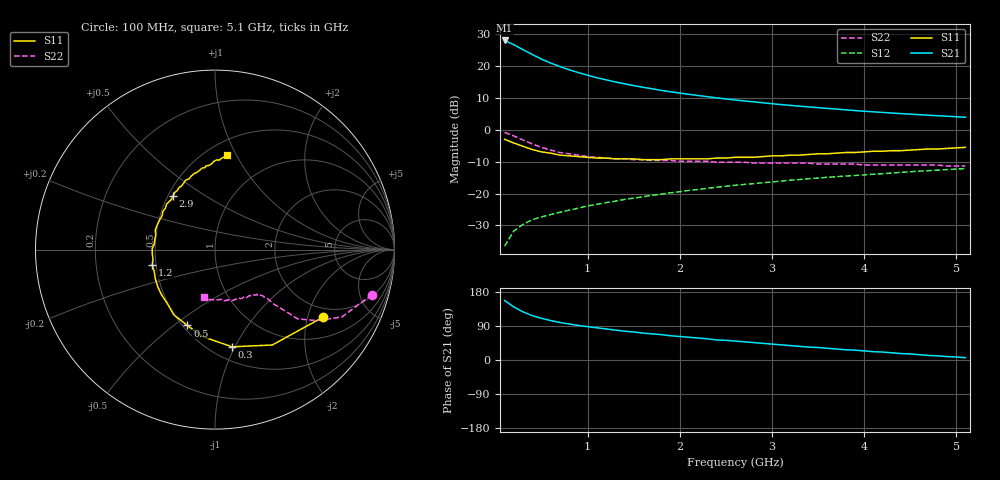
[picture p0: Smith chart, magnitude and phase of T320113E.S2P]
!AT-32011
!S PARAMETERS at Vce=2.7 V  Ic=10mA.  LAST UPDATED 01-05-95
# ghz s ma r 50
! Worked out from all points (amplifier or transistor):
!   51 points, 100 MHz to 5.1 GHz, reference 50 ohm
!   highest |S21| = 28.0 dB at 100 MHz (marker M1)
!   |S21| within 3 dB of that: start of sweep to 306.8 MHz
!   unconditionally stable (mu >= 1): 1.418 GHz to 4.913 GHz
!   at 900 MHz: K = 0.87, MSG = 21.2 dB, |S12| = -24.6 dB
!   at 2.6 GHz: K = 1.08, MAG = 11.6 dB, |S12| = -17.4 dB
!   at 5.1 GHz: K = 0.98, MSG = 8.0 dB, |S12| = -12.2 dB
!   S11 on the Smith chart (normalised r, x): 100 MHz: 1.65, -2.51; 300 MHz: 0.63, -0.97; 500 MHz: 0.53, -0.56; 1.2 GHz: 0.48, -0.10; 2.9 GHz: 0.53, +0.37; 5.1 GHz: 0.62, +0.91
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0.1  0.71 -32.0  25.07 157.0  0.015 75.0  0.91 -16.0
0.2  0.62 -59.0  21.49 140.0  0.026 65.0  0.8 -28.0
0.3  0.55 -80.0  17.96 127.0  0.033 59.0  0.69 -35.0
0.4  0.49 -98.0  15.1 117.0  0.039 56.0  0.6 -40.0
0.5  0.45 -110.0  12.8 110.0  0.043 55.0  0.53 -41.0
0.6  0.43 -122.0  11.1 104.0  0.047 54.0  0.48 -42.0
0.7  0.4 -132.0  9.78 99.0  0.051 54.0  0.44 -43.0
0.8  0.39 -140.0  8.71 95.0  0.055 55.0  0.42 -43.0
0.9  0.38 -147.0  7.86 91.0  0.059 55.0  0.4 -43.0
1  0.37 -154.0  7.15 88.0  0.064 55.0  0.38 -44.0
1.2  0.36 -166.0  6.06 82.0  0.072 56.0  0.36 -45.0
1.4  0.35 -176.0  5.25 76.0  0.081 56.0  0.35 -47.0
1.6  0.34 175.0  4.64 71.0  0.089 56.0  0.34 -48.0
1.8  0.34 166.0  4.14 67.0  0.098 55.0  0.33 -50.0
1.9  0.35 162.0  3.94 64.0  0.103 55.0  0.33 -52.0
2.1  0.35 155.0  3.59 60.0  0.112 54.0  0.32 -54.0
2.4  0.36 144.0  3.16 53.0  0.126 53.0  0.31 -58.0
2.6  0.37 137.0  2.93 50.0  0.135 52.0  0.31 -61.0
2.9  0.38 128.0  2.65 44.0  0.148 49.0  0.3 -65.0
3.5  0.42 113.0  2.22 33.0  0.175 45.0  0.29 -74.0
4.3  0.47 96.0  1.83 19.0  0.21 39.0  0.28 -86.0
5.1  0.53 83.0  1.57 6.0  0.246 32.0  0.27 -103.0
